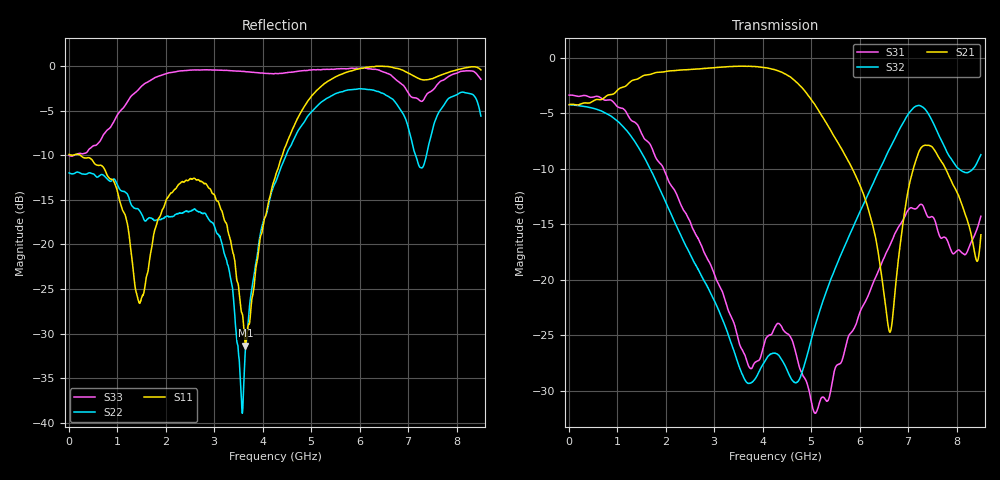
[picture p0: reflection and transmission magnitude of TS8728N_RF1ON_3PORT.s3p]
!Created with skrf (http://scikit-rf.org).
# GHz S RI R 50.0
!freq ReS11 ImS11 ReS12 ImS12 ReS13 ImS13
! ReS21 ImS21 ReS22 ImS22 ReS23 ImS23
! ReS31 ImS31 ReS32 ImS32 ReS33 ImS33
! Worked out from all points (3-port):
!   1601 points, 10 MHz to 8.5 GHz, reference 50 ohm
!   strongest paths, dB at 10 MHz, 2.132 GHz, 4.255 GHz, 6.378 GHz, 8.5 GHz:
!     S21: -4.2, -1.2, -1.1, -17.4, -16.0
!     S32: -4.2, -14.3, -26.6, -10.4, -8.7
!     S31: -3.4, -11.6, -24.3, -19.3, -14.3
!   lowest |S11| = -31.3 dB at 3.645 GHz (marker M1), VSWR 1.06, Z = 47.9 - j1.65 ohm
!   |S11| at or under -10 dB: 68.3406 MHz to 68.41409 MHz (73.49 kHz wide, 0.107 % of centre); 244.1 MHz to 4.407 GHz (4.163 GHz wide, 179 % of centre)
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0.01  -0.3192 0.00687  0.6142 0.0017  0.678 -0.00464
      0.6142 0.00152  -0.2517 0.00708  0.6135 -0.00608
      0.6779 -0.00484  0.6136 -0.00586  -0.315 0.0126
1.755756  0.1086 -0.0365  0.7399 -0.4202  -0.1214 -0.3522
          0.7393 -0.4202  -0.0947 0.0988  -0.1433 -0.2548
          -0.1212 -0.3525  -0.1434 -0.2551  0.7926 -0.3169
2.848844  0.1719 -0.1307  0.4118 -0.7965  -0.1018 -0.074
          0.4113 -0.796  0.0138 0.1433  -0.0888 -0.0316
          -0.102 -0.0739  -0.0889 -0.0317  0.4091 -0.8607
3.644781  -0.0209 -0.0172  0.00963 -0.9146  -0.0349 -0.0285
          0.00954 -0.9146  -0.0228 -0.0121  -0.0117 0.0333
          -0.0349 -0.0285  -0.0115 0.0333  -0.4304 -0.8249
4.255  -0.0313 0.2346  -0.3771 -0.7972  -0.0368 -0.0491
       -0.3783 -0.7966  -0.1641 -0.1476  0.0465 -0.00432
       -0.0369 -0.0488  0.0465 -0.00432  -0.8727 0.2555
5.501969  0.1656 0.8547  -0.4275 -0.0626  0.0301 0.0268
          -0.4278 -0.0623  -0.2942 0.6358  0.1132 0.00633
          0.0301 0.0268  0.1131 0.00639  0.2901 0.917
6.621588  0.2393 0.9604  -0.044 -0.0378  0.1306 -0.057
          -0.044 -0.0378  0.5713 0.3442  0.264 -0.2869
          0.1307 -0.0568  0.2635 -0.2874  0.3571 0.8248
7.152213  0.2319 0.8381  -0.1213 -0.3191  0.0604 -0.1999
          -0.1213 -0.318  0.0703 -0.31  -0.1077 -0.5924
          0.0599 -0.1997  -0.1073 -0.5938  0.1424 0.6479
7.804881  -0.0806 0.912  -0.3021 -0.0407  -0.1058 -0.1065
          -0.303 -0.0413  0.0645 0.6422  -0.3685 -0.0685
          -0.1061 -0.107  -0.3677 -0.0677  -0.1932 0.8419
8.5  -0.2891 0.9066  -0.1024 -0.1226  -0.1935 0.00496
     -0.1021 -0.1223  0.4864 0.1959  -0.2563 0.2597
     -0.193 0.00508  -0.2567 0.2603  -0.3301 0.7757
